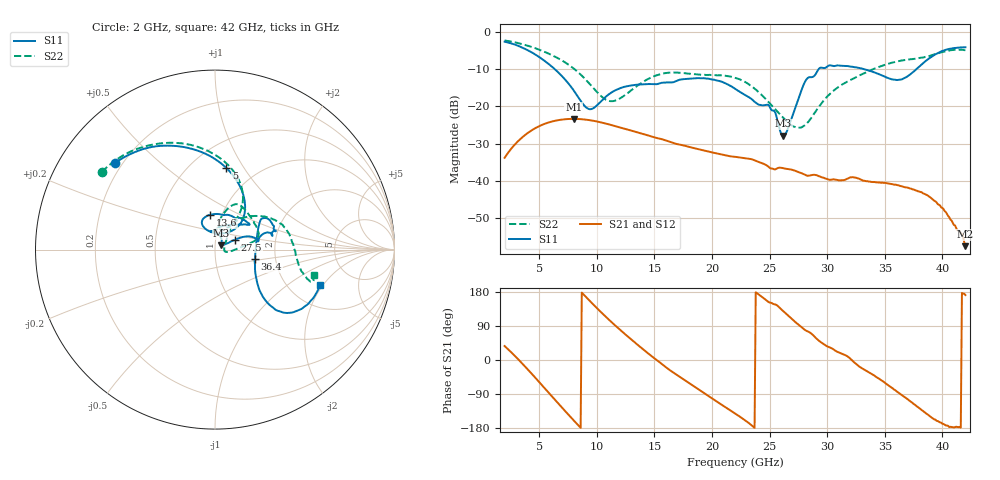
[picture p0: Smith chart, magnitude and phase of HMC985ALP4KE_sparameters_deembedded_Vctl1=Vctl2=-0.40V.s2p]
!s2p File: Measurements: S11, S21, S12, S22
# GHz S dB R 50.0
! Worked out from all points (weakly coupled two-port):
!   401 points, 2 GHz to 42 GHz, reference 50 ohm
!   highest |S21| = -23.36 dB at 8 GHz (marker M1); lowest = -57.5 dB at 42 GHz (marker M2)
!   lowest |S11| = -27.9 dB at 26.2 GHz (marker M3), VSWR 1.08, Z = 53.3 + j2.46 ohm
!   |S11| at or under -10 dB: 6.342 GHz to 29.27 GHz (22.92 GHz wide, 129 % of centre); 33.16 GHz to 37.76 GHz (4.596 GHz wide, 13 % of centre)
!   |S22| runs from -25.8 to -2.3 dB; largest |S21 - S12| = 0.00016
!   S11 on the Smith chart (normalised r, x): 2 GHz: 0.17, +0.36; 5 GHz: 0.73, +0.84; 13.6 GHz: 0.88, +0.35; 27.5 GHz: 1.24, +0.14; 36.4 GHz: 1.56, -0.17; 42 GHz: 2.93, -1.89
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2  -2.65 139.0  -33.80 36.8  -33.80 36.8  -2.33 145.5
3.4  -4.06 112.5  -28.68 -5.1  -28.68 -5.1  -3.21 123.2
5  -6.77 82.0  -25.32 -58.1  -25.32 -58.1  -4.80 98.6
8  -15.76 45.9  -23.36 -159.5  -23.37 -159.5  -9.86 61.0
8.7  -18.96 56.0  -23.46 177.8  -23.46 177.8  -11.77 56.5
9.6  -20.66 90.8  -23.82 149.5  -23.82 149.5  -14.72 55.4
11.1  -16.66 117.2  -24.88 105.0  -24.89 105.0  -18.57 70.3
13.6  -14.17 98.5  -27.06 38.7  -27.06 38.7  -14.30 78.1
15.4  -13.90 73.6  -28.63 -4.6  -28.64 -4.6  -11.47 68.3
19.4  -12.51 36.0  -31.93 -89.2  -31.94 -89.2  -11.56 34.7
22  -15.25 53.4  -33.55 -140.7  -33.58 -140.7  -12.33 14.5
25  -20.04 93.8  -36.48 151.7  -36.50 151.7  -19.16 -0.4
26.2  -27.91 34.9  -36.60 128.6  -36.61 128.6  -23.11 -10.9
27.5  -18.06 26.2  -37.63 93.3  -37.64 93.2  -25.77 0.2
28.1  -13.28 19.1  -38.39 78.8  -38.40 78.9  -25.01 19.1
28.7  -12.15 11.6  -38.41 67.7  -38.42 67.8  -22.73 35.1
31  -9.06 22.2  -39.85 20.2  -39.87 20.0  -14.75 54.2
33.3  -10.11 33.4  -40.02 -26.5  -40.01 -26.6  -11.01 41.5
35.4  -12.52 11.8  -40.76 -68.9  -40.77 -68.8  -8.50 25.5
36.4  -12.82 -13.4  -41.41 -90.8  -41.39 -90.7  -7.73 17.0
39.5  -5.91 -43.2  -45.78 -160.6  -45.80 -160.1  -5.87 -14.9
42  -4.15 -18.7  -57.52 171.4  -57.62 172.3  -4.92 -14.5
